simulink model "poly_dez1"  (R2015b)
settings: Solver=VariableStepAuto  StartTime=0.0  StopTime=10.0  RelTol=1e-3
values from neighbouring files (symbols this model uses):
  g = firpolyphase(hdez, M)    [poly_dez_1.m]    (also in poly_dez_2.m; poly_interp_1.m = firpolyphase(hint, L); poly_interp_2.m = firpolyphase(hint, L))
  hdez = fir1(nord2, 1/M)    [poly_dez_1.m]    (also in poly_dez_2.m)
  hTP = fir1(nord, 2*fp/fs)    [dezimier_2.m]    (also in dezimier_3.m; frac_delay_1.m = fir1(nord, fp*2); frac_delay_2.m = fir1(nord, fp*2); lagrange_3.m = fir1(40, 0.5))
  Ts = 1/fs    (= 5e-05)    [basisband_1.m]    (also in basisband_2.m = 5e-06; dezimier_1.m = 0.0005; dezimier_11.m = 0.0005; dezimier_2.m = 0.0005)
libraries: simulink x1

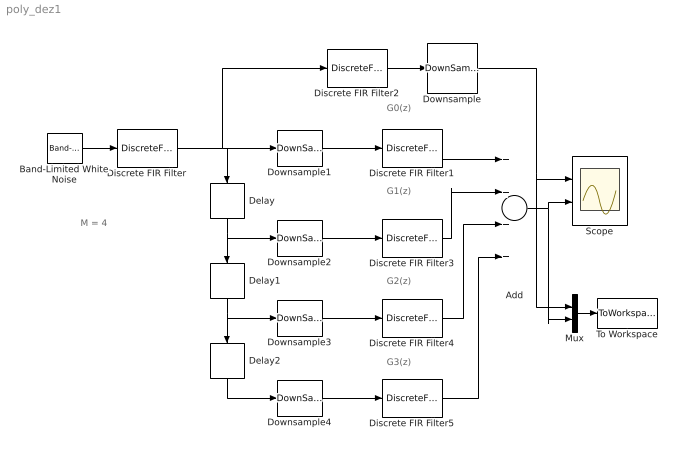
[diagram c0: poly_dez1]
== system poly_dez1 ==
  note: G3(z)
  note: G2(z)
  note: G1(z)
  note: G0(z)
  note: M = 4
  Add : Sum  Inputs=++++
  Band-Limited White Noise : simulink/Sources/Band-Limited White Noise  Cov=Ts  Ts=Ts  seed=[23341]
  Delay : Delay  DelayLength=1
  Delay1 : Delay  DelayLength=1
  Delay2 : Delay  DelayLength=1
  Discrete FIR Filter : DiscreteFir  Coefficients=hTP
  Discrete FIR Filter1 : DiscreteFir  Coefficients=g(1,:)
  Discrete FIR Filter2 : DiscreteFir  Coefficients=hdez
  Discrete FIR Filter3 : DiscreteFir  Coefficients=g(2,:)
  Discrete FIR Filter4 : DiscreteFir  Coefficients=g(3,:)
  Discrete FIR Filter5 : DiscreteFir  Coefficients=g(4,:)
  Downsample{,1..4} (5 alike) : DownSample  N=4  RateOptions=Allow multirate processing
  Mux : Mux  Inputs=2
  Scope : Scope  NumInputPorts=2
  To Workspace : ToWorkspace  VariableName=y  SaveFormat=Timeseries  SampleTime=-1
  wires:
  Band-Limited White Noise/1 -> Discrete FIR Filter/1
  Discrete FIR Filter/1 -> Downsample1/1, Discrete FIR Filter2/1, Delay/1
  Downsample1/1 -> Discrete FIR Filter1/1
  Discrete FIR Filter2/1 -> Downsample/1
  Downsample/1 -> Mux/1, Scope/1
  Downsample2/1 -> Discrete FIR Filter3/1
  Downsample3/1 -> Discrete FIR Filter4/1
  Downsample4/1 -> Discrete FIR Filter5/1
  Delay/1 -> Delay1/1, Downsample2/1
  Delay1/1 -> Delay2/1, Downsample3/1
  Delay2/1 -> Downsample4/1
  Discrete FIR Filter1/1 -> Add/1
  Discrete FIR Filter3/1 -> Add/2
  Discrete FIR Filter4/1 -> Add/3
  Discrete FIR Filter5/1 -> Add/4
  Add/1 -> Mux/2, Scope/2
  Mux/1 -> To Workspace/1
